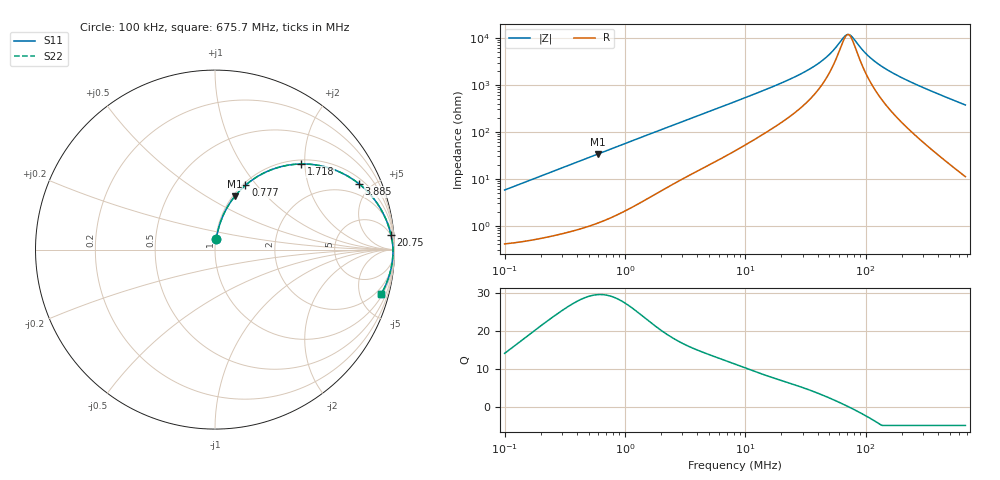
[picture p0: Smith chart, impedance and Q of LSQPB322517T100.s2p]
! LSQPB322517T100  S-PARAMETER MODEL  ( General Type )
! Model Generated by TAIYO YUDEN Corporation (http://www.ty-top.com)
! Version 3.0
! TAIYO YUDEN Control No. 140131NC14SB-FKC
! Copyright(c) 2008 TAIYO YUDEN CO.,LTD. All Rights Reserved.
! Product Description (link to TY-COMPAS)
! https://ds.yuden.co.jp/TYCOMPAS/or/detail?pn=LSQPB322517T100K&u=M
! Products Name : Inductors
! Characteristics :
!  Inductance : 10 uH , SRF(min) : 70 MHz , DC Resistance(max) : 0.42 Ohm
!  Rated Current : Saturation :900 mA , Temp Rise : 700 mA (40 degC)
!  Case Size : 3.2 x 2.5 / 0.126 x 0.098 [mm/inch] , Thickness : 1.7 / 0.068 [mm/inch]
!  (Conditions: Temperature = 25 degC , DC Bias Current/Voltage = 0A / 0V)
! External Node Assignments :
!  1  o---GGG---o  2
! GND o---------o GND
! Frequency Range : 0.1MHz  -  675.68652MHz  [ 402 STEP ]
# MHz S RI R 50
! Freq[MHz].  S11 Real  S11 Imag  S21 Real  S21 Imag  S12 Real  S12 Imag  S22 Real  S22 Imag
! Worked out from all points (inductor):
!   401 points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, 100 kHz to 675.7 MHz, reference 50 ohm
!   read as one part in series: L = 9.15 uH near 104.5 kHz
!   highest Q = 29.5 at 596.4 kHz (marker M1), where L = 9 uH
!   self-resonance near 71.31 MHz
!   S11 on the Smith chart (normalised r, x): 100 kHz: 1.01, +0.12; 777 kHz: 1.03, +0.88; 1.718 MHz: 1.09, +1.92; 3.885 MHz: 1.28, +4.23; 20.75 MHz: 4, +23; 675.7 MHz: 1.22, -7.47
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0.1  0.00736 0.057  0.9926 -0.057  0.9926 -0.057  0.00736 0.057
0.221145  0.0211 0.1231  0.9789 -0.1231  0.9789 -0.1231  0.0211 0.1231
0.438008  0.0654 0.2303  0.9346 -0.2303  0.9346 -0.2303  0.0654 0.2303
0.59638  0.1103 0.2968  0.8897 -0.2968  0.8897 -0.2968  0.1103 0.2968
0.776991  0.1698 0.3586  0.8302 -0.3586  0.8302 -0.3586  0.1698 0.3586
1.207544  0.3217 0.4479  0.6783 -0.4479  0.6783 -0.4479  0.3217 0.4479
1.718276  0.4803 0.477  0.5197 -0.477  0.5197 -0.477  0.4803 0.477
1.918513  0.5316 0.4752  0.4684 -0.4752  0.4684 -0.4752  0.5316 0.4752
3.884582  0.8025 0.3662  0.1975 -0.3662  0.1975 -0.3662  0.8025 0.3662
8.403244  0.9364 0.203  0.0636 -0.203  0.0636 -0.203  0.9364 0.203
20.74894  0.9801 0.0836  0.0199 -0.0836  0.0199 -0.0836  0.9801 0.0836
36.00435  0.9883 0.0405  0.0117 -0.0405  0.0117 -0.0405  0.9883 0.0405
47.95365  0.9904 0.0226  0.00964 -0.0226  0.00964 -0.0226  0.9904 0.0226
54.73535  0.991 0.015  0.00904 -0.015  0.00904 -0.015  0.991 0.015
66.74783  0.9915 0.00377  0.00847 -0.00377  0.00847 -0.00377  0.9915 0.00377
71.31161  0.9916 7.8e-05  0.00836 -7.8e-05  0.00836 -7.8e-05  0.9916 7.8e-05
77.88569  0.9917 -0.00486  0.00828 0.00486  0.00828 0.00486  0.9917 -0.00486
94.97886  0.9917 -0.0162  0.00832 0.0162  0.00832 0.0162  0.9917 -0.0162
110.8275  0.9914 -0.0255  0.0086 0.0255  0.0086 0.0255  0.9914 -0.0255
157.702  0.9898 -0.0492  0.0102 0.0492  0.0102 0.0492  0.9898 -0.0492
292.361  0.9806 -0.1071  0.0194 0.1071  0.0194 0.1071  0.9806 -0.1071
675.6865  0.9268 -0.246  0.0732 0.246  0.0732 0.246  0.9268 -0.246
